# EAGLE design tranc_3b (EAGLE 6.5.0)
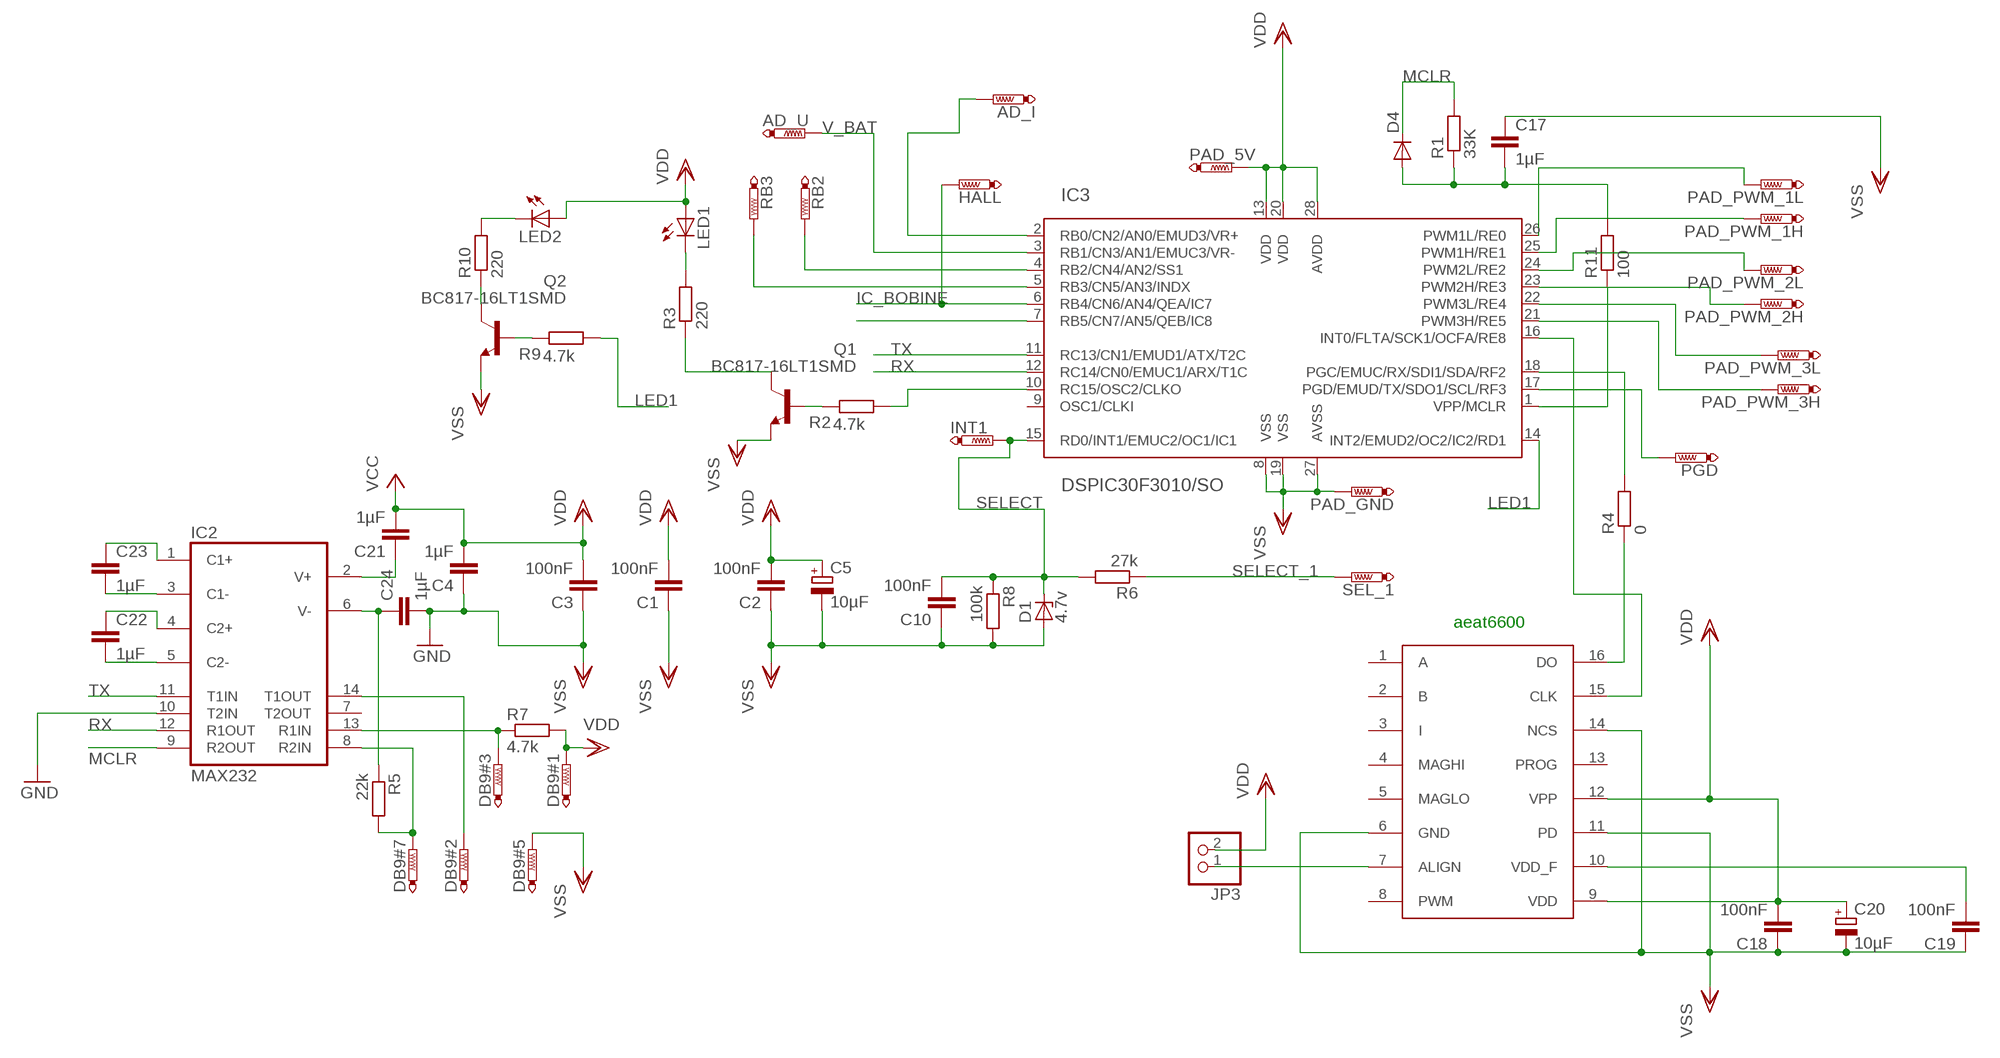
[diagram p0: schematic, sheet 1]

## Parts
AD_I  PTR1TP20SQ  [TP20SQ]
AD_U  PTR1TP20SQ  [TP20SQ]
C1  100nF  C-EUC0805K  [C0805K]
C2  100nF  C-EUC0805K  [C0805K]
C3  100nF  C-EUC0805K  [C0805K]
C4  1µF  C-EUC0805K  [C0805K]
C5  10µF  CPOL-EUSMCB  [SMC_B]
C10  100nF  C-EUC0805K  [C0805K]
C17  1µF  C-EUC0805K  [C0805K]
C18  100nF  C-EUC0805K  [C0805K]
C19  100nF  C-EUC0805K  [C0805K]
C20  10µF  CPOL-EUSMCB  [SMC_B]
C21  1µF  C-EUC0805K  [C0805K]
C22  1µF  C-EUC0805K  [C0805K]
C23  1µF  C-EUC0805K  [C0805K]
C24  1µF  C-EUC0805K  [C0805K]
D1  4.7v  ZENER-DIODESOD80C  [SOD80C]
D4  DIODE-MINIMELF  [MINIMELF]
DB9#1  PTR1TP20SQ  [TP20SQ]
DB9#2  PTR1TP20SQ  [TP20SQ]
DB9#3  PTR1TP20SQ  [TP20SQ]
DB9#5  PTR1TP20SQ  [TP20SQ]
DB9#7  PTR1TP20SQ  [TP20SQ]
HALL  PTR1TP20SQ  [TP20SQ]
IC2  MAX232  [SO16]
IC3  DSPIC30F3010/SO  [SO-28W]
INT1  PTR1TP16SQ  [TP16SQ]
JP3  PINHD-1X2  [1X02]
LED1  LEDCHIPLED_1206  [CHIPLED_1206]
LED2  LEDCHIPLED_1206  [CHIPLED_1206]
PAD_5V  PTR1TP20SQ  [TP20SQ]
PAD_GND  PTR1TP20SQ  [TP20SQ]
PAD_PWM_1H  PTR1TP20SQ  [TP20SQ]
PAD_PWM_1L  PTR1TP20SQ  [TP20SQ]
PAD_PWM_2H  PTR1TP08R  [TP08R]
PAD_PWM_2L  PTR1TP08R  [TP08R]
PAD_PWM_3H  PTR1TP08R  [TP08R]
PAD_PWM_3L  PTR1TP08R  [TP08R]
PGD  PTR1TP10SQ  [TP10SQ]
Q1  BC817-16LT1SMD  [SOT23-BEC]
Q2  BC817-16LT1SMD  [SOT23-BEC]
R1  33K  R-EU_M1206  [M1206]
R2  4.7k  R-EU_M0805  [M0805]
R3  220  R-EU_M0805  [M0805]
R4  0  R-EU_R0805W  [R0805W]
R5  22k  R-EU_M1206  [M1206]
R6  27k  R-EU_M1206  [M1206]
R7  4.7k  R-EU_M1206  [M1206]
R8  100k  R-EU_M0805  [M0805]
R9  4.7k  R-EU_M0805  [M0805]
R10  220  R-EU_M0805  [M0805]
R11  100  R-EU_M0805  [M0805]
RB2  PTR1TP10SQ  [TP10SQ]
RB3  PTR1TP10SQ  [TP10SQ]
SEL_1  PTR1TP20SQ  [TP20SQ]
U$3  AVAGO_AEAT-6600TSSOP16  [AVAGO_TSSOP16]

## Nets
IC_BOBINE: HALL.TP IC3.6(RB4/CN6/AN4/QEA/IC7)
LED1: IC3.14(INT2/EMUD2/OC2/IC2/RD1) R9.1
MCLR: D4.C IC2.9(R2OUT) R1.2
MCLR1: IC3.1(VPP/MCLR) R11.1
N$1: R4.1 U$3.16(DO)
N$2: IC3.21(PWM3H/RE5) PAD_PWM_3H.TP
N$3: IC3.16(INT0/FLTA/SCK1/OCFA/RE8) U$3.15(CLK)
N$4: IC3.22(PWM3L/RE4) PAD_PWM_3L.TP
N$5: Q1.B R2.2
N$6: Q1.C R3.1
N$7: IC3.7(RB5/CN7/AN5/QEB/IC8)
N$9: C17.2 D4.A R1.1 R11.2
N$10: IC3.23(PWM2H/RE3) PAD_PWM_2H.TP
N$11: IC3.25(PWM1H/RE1) PAD_PWM_1H.TP
N$12: IC3.26(PWM1L/RE0) PAD_PWM_1L.TP
N$13: IC3.24(PWM2L/RE2) PAD_PWM_2L.TP
N$14: JP3.1 U$3.7(ALIGN)
N$15: IC3.17(PGD/EMUD/TX/SDO1/SCL/RF3) PGD.TP
N$17: IC3.18(PGC/EMUC/RX/SDI1/SDA/RF2) R4.2
N$18: IC3.10(RC15/OSC2/CLKO) R2.1
N$19: IC3.5(RB3/CN5/AN3/INDX) RB3.TP
N$20: IC3.4(RB2/CN4/AN2/SS1) RB2.TP
N$21: Q2.B R9.2
N$22: Q2.C R10.1
N$23: LED1.C R3.2
N$24: LED2.C R10.2
N$27: C23.1 IC2.1(C1+)
N$28: C23.2 IC2.3(C1-)
N$29: C22.2 IC2.5(C2-)
N$30: AD_I.TP IC3.2(RB0/CN2/AN0/EMUD3/VR+)
N$31: C19.2 U$3.10(VDD_F)
N$32: C22.1 IC2.4(C2+)
N$33: C21.1 IC2.2(V+)
N$34: C24.1 IC2.6(V-) R5.1
N$35: DB9#3.TP IC2.13(R1IN) R7.1
N$36: DB9#2.TP IC2.14(T1OUT)
N$37: DB9#7.TP IC2.8(R2IN) R5.2
RX: IC2.12(R1OUT) IC3.12(RC14/CN0/EMUC1/ARX/T1C)
SELECT: C10.2 D1.C IC3.15(RD0/INT1/EMUC2/OC1/IC1) INT1.TP R6.2 R8.1
SELECT_1: R6.1 SEL_1.TP
TX: IC2.11(T1IN) IC3.11(RC13/CN1/EMUD1/ATX/T2C)
V_BAT: AD_U.TP IC3.3(RB1/CN3/AN1/EMUC3/VR-)
VDD: C1.2 C2.2 C3.2 C4.2 C5.+ C18.2 C20.+ C21.2 DB9#1.TP IC3.13(VDD) IC3.20(VDD) IC3.28(AVDD) JP3.2 LED1.A LED2.A PAD_5V.TP R7.2 U$3.9(VDD) U$3.12(VPP) ; supply symbol labelled VCC
VSS: C1.1 C2.1 C3.1 C4.1 C5.- C10.1 C17.1 C18.1 C19.1 C20.- C24.2 D1.A DB9#5.TP IC2.10(T2IN) IC3.8(VSS) IC3.19(VSS) IC3.27(AVSS) PAD_GND.TP Q1.E Q2.E R8.2 U$3.6(GND) U$3.11(PD) U$3.14(NCS) ; supply symbol labelled GND
Unconnected: IC2.7(T2OUT) IC3.9(OSC1/CLKI) U$3.1(A) U$3.2(B) U$3.3(I) U$3.4(MAGHI) U$3.5(MAGLO) U$3.8(PWM) U$3.13(PROG)

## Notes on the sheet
- aeat6600

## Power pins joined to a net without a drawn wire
VDD: IC2.16(VCC)
VSS: IC2.15(GND)

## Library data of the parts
AD_I AD_U DB9#1-DB9#3 DB9#5 DB9#7 HALL INT1 PAD_5V PAD_GND PAD_PWM_1H PAD_PWM_1L PAD_PWM_2H PAD_PWM_2L PAD_PWM_3H PAD_PWM_3L PGD RB2 RB3 SEL_1 = testpad:PTR1: TEST PIN
C1-C4 C10 C17-C19 C21-C24 = rcl:C-EU: CAPACITOR, European symbol
C5 C20 = rcl:CPOL-EU: POLARIZED CAPACITOR, European symbol
D1 = diode:ZENER-DIODE: Z-Diode
D4 = diode:DIODE-: DIODE
IC2 = maxim:MAX232: RS232 TRANSCEIVER
IC3 = microchip-dspic:DSPIC30F3010: dsPIC Motion Controller DSC
JP3 = pinhead:PINHD-1X2: PIN HEADER
LED1 LED2 = led:LED: LED
Q1 Q2 = transistor-npn:BC817*: NPN Transistor
R1-R11 = rcl:R-EU_: RESISTOR, European symbol
U$3 = aeat_6600_1:AVAGO_AEAT-6600

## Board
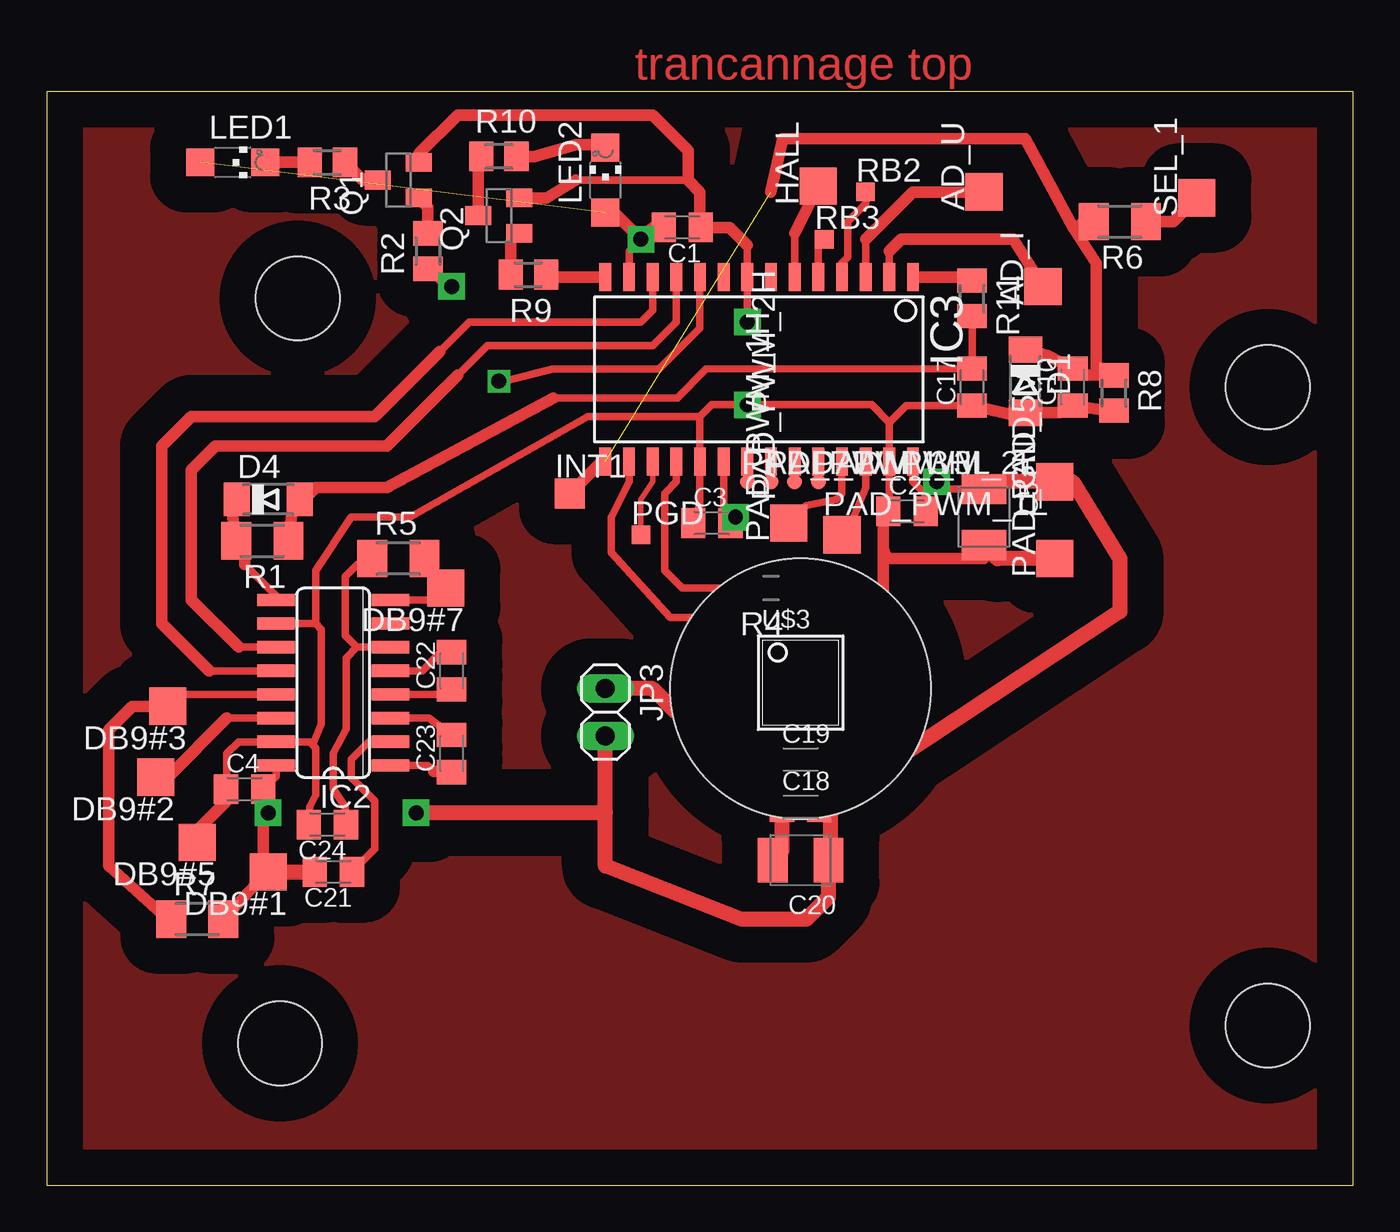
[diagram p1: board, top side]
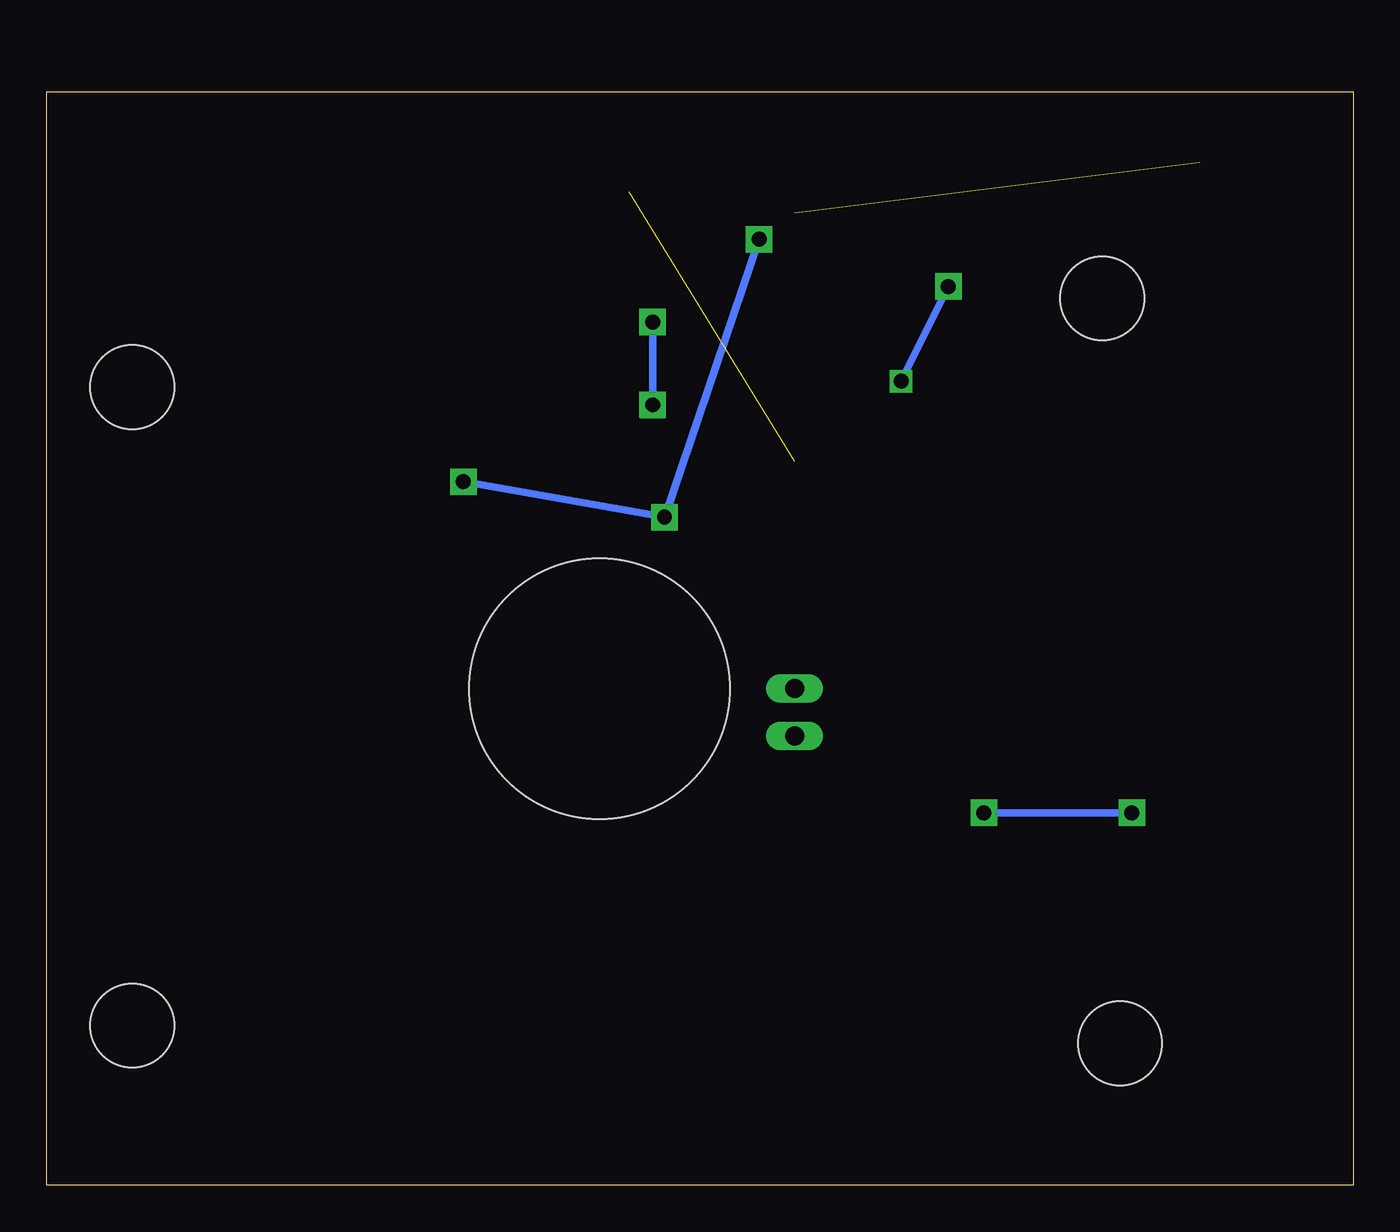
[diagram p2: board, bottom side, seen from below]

Size 70.16 x 58.73 mm. Coordinates in mm from the lower left corner, seen from the top.
Outline: 0,0 70.16,0 70.16,58.73 0,58.73 0,0
Copper layers (1*16): Top 0.035mm / dielectric 1.5mm / Bottom 0.035mm
Design rules "default": minimum track width 10mil, minimum drill 24mil, track to track 8mil, track to pad 8mil, pad to pad 8mil, via to via 8mil, smd to smd 8mil, copper to edge 40mil, drill to drill 8mil, minimum pad ring 10mil, minimum via ring 8mil, stop-mask expansion 4mil, vias tented up to drill 0mil, thermal gap 10mil
Holes 14 mm at 40.48,26.66
Holes 4.5 mm at 13.49,47.62 65.56,42.86 12.54,7.62 65.56,8.57

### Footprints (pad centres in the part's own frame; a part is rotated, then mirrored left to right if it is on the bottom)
TP20SQ = smd 2 x 2: TP 0,0
C0805K = smd 1.3 x 1.6: 1 -1,0; 2 1,0
SMC_B = smd 1.6 x 2.4: + -1.5,0; - 1.5,0
SOD80C = smd 1.4 x 1.8: A 1.7,0; C -1.7,0
MINIMELF = smd 1.4 x 1.8: A 1.7,0; C -1.7,0
SO16 = smd 0.66 x 2.032: 1 -4.445,-3.073; 2 -3.175,-3.073; 3 -1.905,-3.073; 4 -0.635,-3.073; 5 0.635,-3.073; 6 1.905,-3.073; 7 3.175,-3.073; 8 4.445,-3.073; 9 4.445,3.073; 10 3.175,3.073; 11 1.905,3.073; 12 0.635,3.073; 13 -0.635,3.073; 14 -1.905,3.073; 15 -3.175,3.073; 16 -4.445,3.073
SO-28W = smd 0.635 x 1.524: 1 -7.62,-4.953; 2 -6.35,-4.953; 3 -5.08,-4.953; 4 -3.81,-4.953; 5 -2.54,-4.953; 6 -1.27,-4.953; 7 0,-4.953; 8 1.27,-4.953; 9 2.54,-4.953; 10 3.81,-4.953; 11 5.08,-4.953; 12 6.35,-4.953; 13 7.62,-4.953; 14 8.89,-4.953; 15 8.89,4.953; 16 7.62,4.953; 17 6.35,4.953; 18 5.08,4.953; 19 3.81,4.953; 20 2.54,4.953; 21 1.27,4.953; 22 0,4.953; 23 -1.27,4.953; 24 -2.54,4.953; 25 -3.81,4.953; 26 -5.08,4.953; 27 -6.35,4.953; 28 -7.62,4.953
TP16SQ = smd 1.6 x 1.6: TP 0,0
1X02 = drill 1.016 long: 1 -1.27,0; 2 1.27,0
CHIPLED_1206 = smd 1.5 x 1.5: A 0,-1.75; C 0,1.75
TP08R = smd 0.8 x 0.8: TP 0,0
TP10SQ = smd 1 x 1: TP 0,0
SOT23-BEC = smd 1 x 1.4: B -0.95,-1.1; C 0,1.1; E 0.95,-1.1
M1206 = smd 1.6 x 2: 1 -1.4,0; 2 1.4,0
M0805 = smd 1.3 x 1.6: 1 -0.95,0; 2 0.95,0
R0805W = smd 1.5 x 1: 1 -1.052,0; 2 1.052,0
AVAGO_TSSOP16 = smd 0.305 x 0.991: 1 -2.275,-2.918; 2 -1.625,-2.918; 3 -0.975,-2.918; 4 -0.325,-2.918; 5 0.325,-2.918; 6 0.975,-2.918; 7 1.625,-2.918; 8 2.275,-2.918; 9 2.275,2.918; 10 1.625,2.918; 11 0.975,2.918; 12 0.325,2.918; 13 -0.325,2.918; 14 -0.975,2.918; 15 -1.625,2.918; 16 -2.275,2.918

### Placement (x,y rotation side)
AD_I  53.49,48.26 90 top
AD_U  50.32,53.34 90 top
C1  34.12,51.43 180 top
C2  46.19,36.19 0 top
C3  35.71,35.55 0 top
C4  10.63,21.27 0 top
C5  50.32,35.87 270 top
C10  55.08,42.86 90 top
C17  49.68,42.86 90 top
C18  40.48,20.32 0 top
C19  40.48,22.86 0 top
C20  40.48,17.46 180 top
C21  15.39,16.82 180 top
C22  21.74,27.62 90 top
C23  21.74,23.17 90 top
C24  15.08,19.36 180 top
D1  52.54,43.17 270 top
D4  11.9,36.83 0 top
DB9#1  11.9,16.82 180 top
DB9#2  5.87,21.9 180 top
DB9#3  6.5,25.71 180 top
DB9#5  8.09,18.41 180 top
DB9#7  21.42,32.06 180 top
HALL  41.43,53.65 90 top
IC2  15.39,26.98 90 top
IC3  38.89,43.81 180 top
INT1  28.09,37.14 0 top
JP3  30,25.39 270 top
LED1  10,54.92 270 top
LED2  30,53.97 0 top
PAD_5V  54.13,37.78 90 top
PAD_GND  54.13,33.65 90 top
PAD_PWM_1H  39.84,35.55 90 top
PAD_PWM_1L  42.7,34.92 0 top
PAD_PWM_2H  40.16,37.78 90 top
PAD_PWM_2L  41.43,37.78 0 top
PAD_PWM_3H  37.62,37.78 0 top
PAD_PWM_3L  38.89,37.78 0 top
PGD  31.9,34.92 0 top
Q1  18.88,53.97 90 top
Q2  24.28,52.06 90 top
R1  11.58,34.6 180 top
R2  20.47,50.16 90 top
R3  15.08,54.92 180 top
R4  38.89,32.06 180 top
R5  18.88,33.65 0 top
R6  57.62,51.75 180 top
R7  8.09,14.28 0 top
R8  57.3,42.54 270 top
R9  25.87,48.89 180 top
R10  24.28,55.24 0 top
R11  49.68,47.62 270 top
RB2  43.97,53.34 0 top
RB3  41.74,50.8 0 top
SEL_1  61.75,53.02 90 top
U$3  40.48,26.98 270 top

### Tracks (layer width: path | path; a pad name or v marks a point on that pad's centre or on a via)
IC_BOBINE
  Top 0.406: IC3.6 40.16,51.11
  Top 0.61: 40.16,51.11 HALL.TP
LED1
  Top 0.61: IC3.14 26.95,48.76 R9.1
MCLR
  Top 0.406: 10,35.88 10,36.83 10,36.62 D4.C | IC2.9 12.32,31.64 10.63,33.33 | 10.63,34.6 R1.2
  Top 0.61: R1.2 10,35.88 | 10.63,33.33 10.63,34.6
MCLR1
  Top 0.406: 49.49,48.76 R11.1
  Top 0.61: IC3.1 49.49,48.76
N$1
  Top 0.406: R4.1 40.59,32.06 U$3.16
N$2
  Top 0.406: PAD_PWM_3H.TP IC3.21
N$3
  Top 0.254: U$3.15 41.07,28.61 40.79,28.89
  Top 0.406: 40.79,28.89 39.2,30.48 33.49,30.48 30.31,33.97 30.31,35.87 31.27,37.78 IC3.16
N$4
  Top 0.406: PAD_PWM_3L.TP IC3.22
N$5
  Top 0.61: R2.2 20.47,52.53 Q1.B
N$6
  Top 0.61: Q1.C 16.98,53.97 R3.1
N$8
  pour Top (isolate 1.93): 0.47,58.73 70.32,58.73 70.32,0.31 0.15,0.31
N$9
  Top 0.406: R11.2 C17.2 35.39,43.81 33.85,42.27 27.19,42.27 | 12.58,34.65 R1.1 | 13.17,35.99 D4.A 13.81,36.83
  Top 0.61: R1.1 13.17,35.99 | 27.19,42.27 18.25,37.46 14.44,37.46 13.81,36.83
N$10
  Top 0.406: PAD_PWM_2H.TP IC3.23
N$11
  Top 0.406: IC3.25 42.7,37.14 42.38,36.83 40.79,36.51 PAD_PWM_1H.TP
N$12
  Top 0.406: IC3.26 43.97,37.46 43.33,35.87 PAD_PWM_1L.TP
N$13
  Top 0.406: PAD_PWM_2L.TP IC3.24
N$14
  Top 0.254: U$3.7 35.43,25.36 35.39,25.39
  Top 0.406: 35.39,25.39 33.81,25.39
  Top 0.813: 33.81,25.39 32.54,26.66 JP3.1
N$15
  Top 0.305: IC3.17 32.54,37.78 31.9,36.83 PGD.TP 31.9,34.6
N$17
  Top 0.406: R4.2 34.12,32.06 33.17,33.02 33.17,37.14 33.81,37.78 IC3.18
N$18  (via drill 0.8, 0.8 pad 1.42)
  Top 0.406: IC3.10 35.08,46.03 32.85,43.81 27.14,43.81 24.6,43.17 v24.28,43.17 | v21.74,48.26 21.43,48.26 R2.1
  Bottom 0.406: v24.28,43.17 v21.74,48.26
N$19
  Top 0.406: IC3.5 41.43,50.48 RB3.TP
N$20
  Top 0.406: IC3.4 42.7,49.52 43.02,49.84 43.02,51.75 43.97,52.7 RB2.TP
N$21
  Top 0.406: 24.92,50.65 Q2.B
  Top 0.61: R9.2 24.92,50.65
N$22
  Top 0.406: 23.18,55.09 R10.1
  Top 0.61: Q2.C 23.18,55.09
N$23
  Top 0.61: R3.2 LED1.C
N$24
  Top 0.406: 29.84,55.88 LED2.C
  Top 0.61: R10.2 26.19,55.24 28.41,55.88 29.84,55.88
N$27
  Top 0.406: IC2.1 20.47,22.54 20.79,22.22 | 22.01,22.22 C23.1
  Top 0.61: 20.79,22.22 22.01,22.22
N$28
  Top 0.406: IC2.3 20.52,25.08 C23.2
N$29
  Top 0.406: IC2.5 20.15,27.62 21.11,28.57 22.01,28.57 C22.2
N$30
  Top 0.406: IC3.2 45.24,50.16
  Top 0.61: 45.24,50.16 45.87,50.8 51.91,50.8 AD_I.TP
N$31
  Top 0.254: U$3.10 42.34,25.36 41.43,24.44
  Top 0.406: 41.43,24.44 41.43,22.9 C19.2
N$32
  Top 0.406: IC2.4 22.06,26.35 C22.1
N$33
  Top 0.406: 16.34,16.77 C21.1 17.61,18.05 17.61,20.63 16.34,21.9 16.34,22.86 17.3,23.81 IC2.2
N$34
  Top 0.406: C24.1 16.03,20.32 15.39,21.27 15.39,23.17 16.07,24.49 16.07,28.3 16.66,28.89 | 16.66,28.89 IC2.6 | R5.1 16.66,33.34 16.03,32.7 16.03,29.52 16.66,28.89
N$35
  Top 0.406: IC2.13 7.14,26.35 DB9#3.TP
  Top 0.61: R7.1 6.5,14.28 3.33,17.14 3.33,24.44 4.6,25.71 DB9#3.TP
N$36
  Top 0.406: IC2.14 9.68,25.08 | 6.5,21.9 DB9#2.TP
  Top 0.61: 9.68,25.08 6.5,21.9
N$37
  Top 0.406: IC2.8 21.42,31.43 DB9#7.TP 20.29,33.2 R5.2
RX
  Top 0.406: IC2.12 8.73,27.62 | 21.11,44.76 22.7,46.35 31.9,46.35 32.54,46.98 IC3.12
  Top 0.61: 8.73,27.62 6.18,30.16 6.18,39.68 7.77,41.27 17.61,41.27 21.11,44.76
SELECT  (1 unrouted)
  Top 0.406: 55.4,43.49 54.81,43.49 C10.2 | R6.2 55.52,51.75 55.13,51.36
  Top 0.61: R8.1 56.35,43.49 | 56.35,43.49 55.4,43.49 | D1.C 53.74,44.56 C10.2 | 38.89,53.34 39.52,56.19 52.54,56.19 55.13,51.36 56.35,49.52 56.35,43.49 | IC3.15 29.81,38.86 INT1.TP
SELECT_1
  Top 0.61: R6.1 60.48,51.75 SEL_1.TP
TX
  Top 0.406: IC3.11 33.81,46.35 32.54,45.08 23.65,45.08 22.06,43.49 | 10.31,28.89 IC2.11
  Top 0.61: 22.06,43.49 18.25,39.68 9.04,39.68 7.77,38.41 7.77,31.43 10.31,28.89
V_BAT
  Top 0.406: IC3.3 43.97,50.8
  Top 0.61: 43.97,50.8 46.51,53.34 AD_U.TP
VDD  (via drill 0.8 pad 1.42)  (1 unrouted)
  Top 0.254: U$3.9 43.97,24.71 44.55,24.71 44.92,25.08 44.92,26.35 44.6,26.66 U$3.12
  Top 0.406: IC2.16 12.32,21.96 C4.2 11.63,20.32 11.95,20 v11.9,20 | 11.63,17.09 DB9#1.TP | C18.2 42.06,20.63 | 43.49,21.43 43.65,21.59 43.65,24.39 43.97,24.71 | IC3.20 36.35,36.55 C3.2 v36.98,35.87 | 42.06,17.86 C20.+ | 32.54,51.43 C1.2 | 50.72,37.78 C5.+ 47.78,37.37 | IC3.13 31.27,50.16 v31.9,50.8 | IC3.28 46.51,37.78 47.14,37.14 | 47.14,37.14 47.14,36.24 C2.2 | 47.78,37.37 47.37,37.37 47.14,37.14 | v47.78,37.78 47.78,37.37 | PAD_5V.TP 55.08,37.78
  Top 0.61: 11.63,20.32 11.63,17.09 | 32.54,51.43 v31.9,50.8 30.16,52.54 LED2.A | R7.2 11.26,16.18 DB9#1.TP
  Top 0.813: DB9#1.TP C21.2 | 43.49,21.43 42.06,20.63 42.06,17.86 | PAD_5V.TP 50.72,37.78 | C20.+ 41.98,15.46 40.79,14.28 37.3,14.28 30,17.14 30,20 | 30,20 JP3.2 | 30,20 v19.84,20 | 55.08,37.78 57.62,33.65 57.62,30.79 43.65,21.59
  Bottom 0.406: v19.84,20 v11.9,20 | v31.9,50.8 v36.98,35.87 v47.78,37.78
VSS  (via drill 0.8 pad 1.42)
  Top 0.254: U$3.11 41.43,26.01 | 41.43,26.01 39.84,26.01 U$3.6 | 41.43,26.01 41.43,27.3 42.09,27.96 U$3.14 44.62,27.96 44.92,28.25
  Top 0.406: 9.63,20.59 C4.1 9.68,21.32 9.68,23.17 10.31,23.81 IC2.15 14.12,23.81 14.28,23.65 | 7.46,18.41 DB9#5.TP | 14.28,23.65 14.44,23.49 14.44,20.95 14.12,20.32 14.12,19.41 C24.2 | IC2.10 14.44,30.16 | 14.28,23.65 14.76,24.76 14.76,29.84 14.44,30.16 | 39.84,26.01 39.48,25.64 C19.1 C18.1 | C3.1 35.08,36.55 IC3.19 35.08,41.27 | C17.1 46.14,41.86 45.24,40.95 | 45.24,40.95 IC3.27 45.24,36.24 C2.1 44.92,35.92 | 35.08,41.27 35.71,41.91 v37.62,41.91 44.28,41.91 45.24,40.95 | 39.48,17.96 C20.- | 35.08,41.27 35.07,41.27 29.04,41.27 19.52,35.87 16.34,35.87 14.44,33.02 14.44,30.16 | 37.62,50.48 IC3.8 v37.62,46.35 | 52.48,41.22 D1.A | 54.38,41.48 C10.1 | 57.25,41.54 R8.2 | 45.15,33.74 44.92,34.6 | 28.41,53.97 34.44,53.97 | 35.08,51.48 C1.1
  Top 0.61: 9.63,20.59 7.46,18.41 | 44.92,28.25 44.92,34.6 44.92,35.92 | 37.62,50.48 36.66,51.43 C1.1 | C17.1 52.48,41.22 | D1.A 54.38,41.48 | C10.1 57.25,41.54 | C5.- 50.32,33.65 44.92,33.65 45.01,33.74 45.15,33.74 | Q2.E 26.82,53.02 28.41,53.97 | 35.08,51.48 35.08,53.34 34.44,53.97 34.44,55.56 32.54,57.46 22.06,57.46 19.98,55.39 Q1.E
  Top 0.813: C18.1 39.48,17.96 | PAD_GND.TP 51.04,33.65 C5.-
  Bottom 0.406: v37.62,41.91 v37.62,46.35

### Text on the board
Top: trancannage top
